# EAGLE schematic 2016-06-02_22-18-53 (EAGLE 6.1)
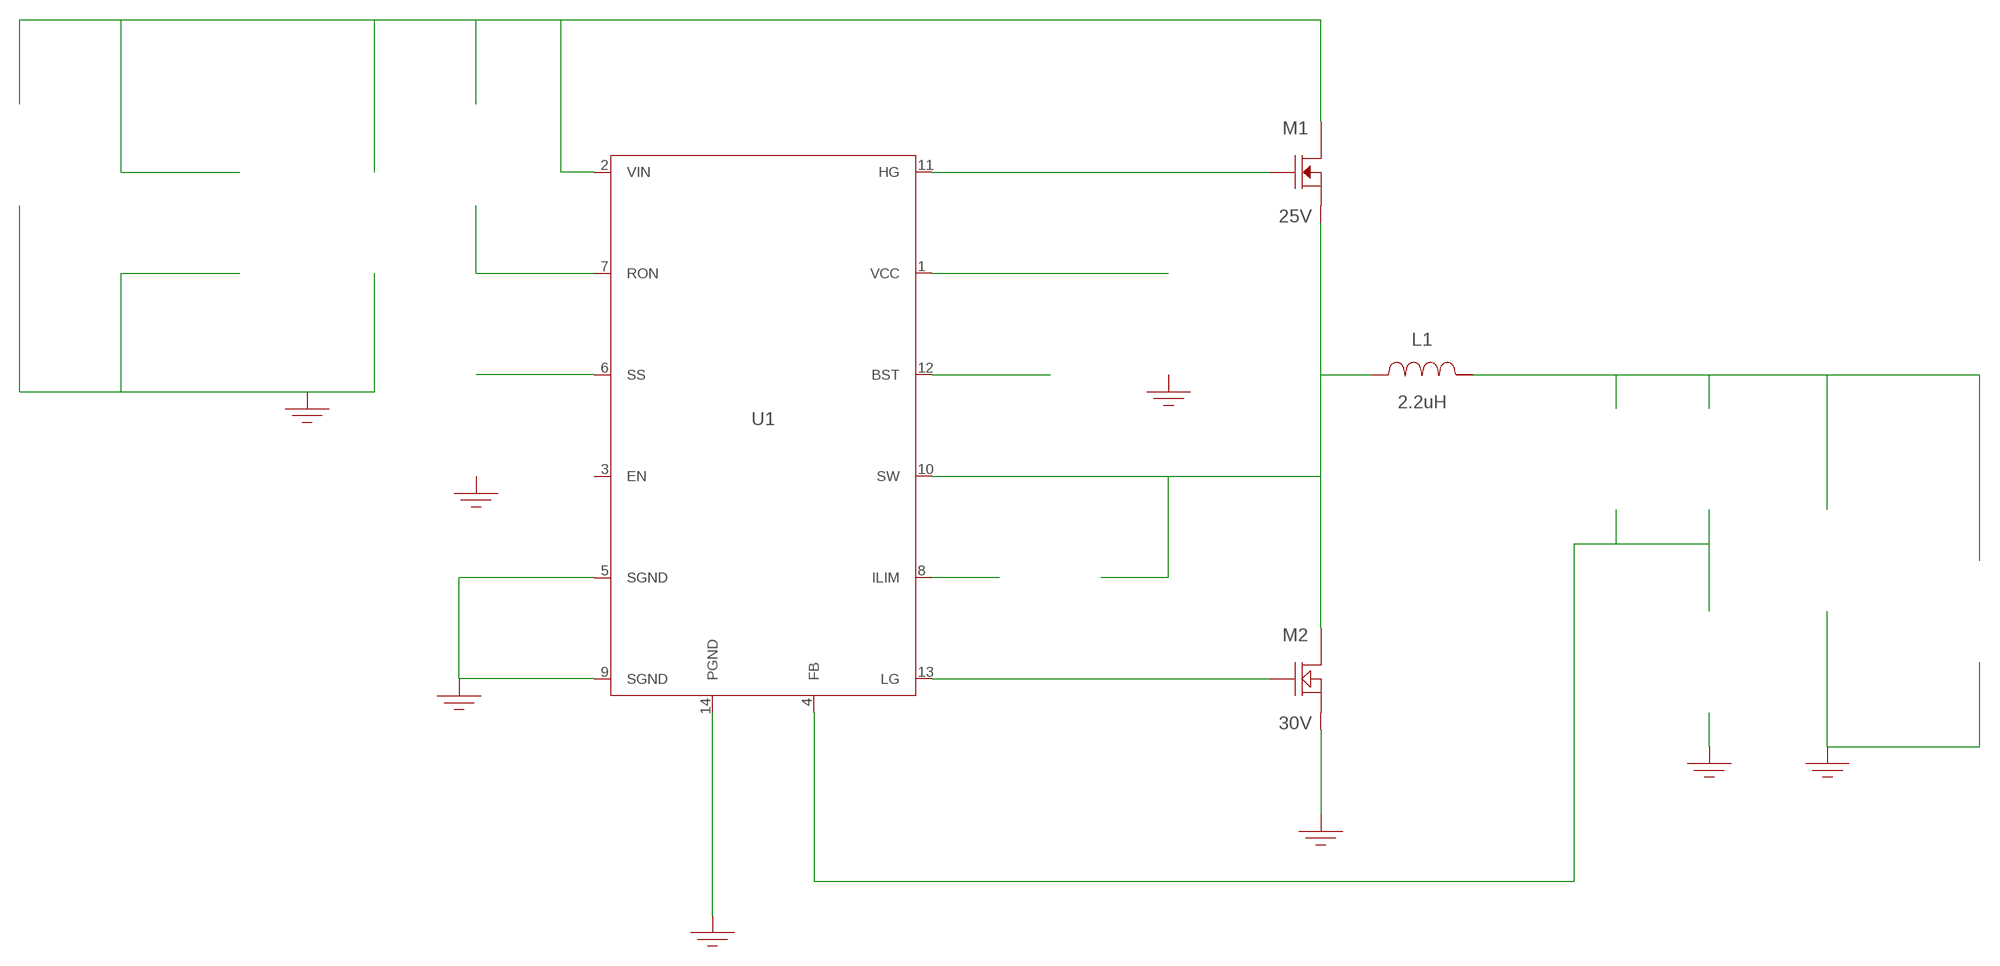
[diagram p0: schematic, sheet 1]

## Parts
CBST  470nF  EMK212B7474KD-TEMK212B7474KD-T  [0805]  (not placed on a sheet)
CBYP  100nF  08053C104KAT2A08053C104KAT2A  [0805]  (not placed on a sheet)
CFF  470pF  C0805C471K5RACTUC0805C471K5RACTU  [0805]  (not placed on a sheet)
CIN  22uF  GRM32ER61E226KE15LGRM32ER61E226KE15L  [1210]  (not placed on a sheet)
CIN_2  22uF  GRM32ER61E226KE15LGRM32ER61E226KE15L  [1210]  (not placed on a sheet)
COUT  220uF  6SVPE220MW6SVPE220MW  [CAPSMT_62_E61]  (not placed on a sheet)
CSS  15nF  CC0805KRX7R9BB153CC0805KRX7R9BB153  [0805]  (not placed on a sheet)
CVCC  1uF  EMK212B7105KG-TEMK212B7105KG-T  [0805]  (not placed on a sheet)
GND1  WB_GND  WB_GNDWB_GND  [WB_GND]
GND2  WB_GND  WB_GNDWB_GND  [WB_GND]
GND3  WB_GND  WB_GNDWB_GND  [WB_GND]
GND4  WB_GND  WB_GNDWB_GND  [WB_GND]
GND5  WB_GND  WB_GNDWB_GND  [WB_GND]
GND6  WB_GND  WB_GNDWB_GND  [WB_GND]
GND7  WB_GND  WB_GNDWB_GND  [WB_GND]
GND8  WB_GND  WB_GNDWB_GND  [WB_GND]
IOUT  WB_CURRENT_LOAD  WB_CURRENT_LOADWB_CURRENT_LOAD  [WB_CURRENT_LOAD]  (not placed on a sheet)
L1  2.2uH  SRP1270-2R2MSRP1270-2R2M  [SRP1270]
M1  25V  CSD16342Q5ACSD16342Q5A  [TRANS_NexFET_Q5A]
M2  30V  CSD17577Q5ACSD17577Q5A  [TRANS_NexFET_Q5A]
RFB1  10k  ERJ-6ENF1002VERJ-6ENF1002V  [0805]  (not placed on a sheet)
RFB2  73.2k  ERJ-6ENF7322VERJ-6ENF7322V  [0805]  (not placed on a sheet)
RILIM  1.05k  ERJ-6ENF1051VERJ-6ENF1051V  [0805]  (not placed on a sheet)
RON  100k  ERJ-6ENF1003VERJ-6ENF1003V  [0805]  (not placed on a sheet)
U1  LM3150MH/NOPB  LM3150MH/NOPBLM3150MH/NOPB  [MXA14A]
VIN  WB_BATTERY  WB_BATTERYWB_BATTERY  [WB_BATTERY]  (not placed on a sheet)

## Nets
0: Cbyp.2@2 Cin.2@2 Cin_2.2@2 Cout.-@2 Css.2@2 Cvcc.2@2 GND1.1 GND2.1 GND3.1 GND4.1 GND5.1 GND6.1 GND7.1 GND8.1 Iout.-@2 M2.1(Source) M2.2(Source) M2.3(Source) Rfb1.2@2 U1.5(SGND) U1.9(SGND) U1.14(PGND) U1.15(DAP) Vin.-@2
1: Css.1@1 U1.6(SS)
2: Cbyp.1@1 Cin.1@1 Cin_2.1@1 M1.5(Drain) M1.6(Drain) M1.7(Drain) M1.8(Drain) M1.9(Drain) Ron.1@1 U1.2(VIN) Vin.+@1
3: Ron.2@2 U1.7(RON)
4: Cff.1@1 Cout.+@1 Iout.+@1 L1.2 Rfb2.1@1
5: Cff.2@2 Rfb1.1@1 Rfb2.2@2 U1.4(FB)
6: Cbst.2@2 L1.1 M1.1(Source) M1.2(Source) M1.3(Source) M2.5(Drain) M2.6(Drain) M2.7(Drain) M2.8(Drain) M2.9(Drain) Rilim.1@1 U1.10(SW)
7: M2.4(Gate) U1.13(LG)
8: M1.4(Gate) U1.11(HG)
9: Cbst.1@1 U1.12(BST)
10: Cvcc.1@1 U1.1(VCC)
11: Rilim.2@2 U1.8(ILIM)
Unconnected: CBST.1 CBST.2 CBYP.1 CBYP.2 CFF.1 CFF.2 CIN.1 CIN.2 CIN_2.1 CIN_2.2 COUT.1(+) COUT.2(-) CSS.1 CSS.2 CVCC.1 CVCC.2 IOUT.1(+) IOUT.2(-) RFB1.1 RFB1.2 RFB2.1 RFB2.2 RILIM.1 RILIM.2 RON.1 RON.2 U1.3(EN) VIN.1(+) VIN.2(-)

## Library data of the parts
CBST = AcceleratedDesigns_Lib:EMK212B7474KD-T; Cap: 4.7E-7; ESR: 0.0; IRMS: 0.0; Manufacturer_Name: Taiyo Yuden; Manufacturer_Part_Number: EMK212B7474KD-T; VDC: 16.0; Vendor: Taiyo Yuden
CBYP = AcceleratedDesigns_Lib:08053C104KAT2A; Cap: 1.0E-7; ESR: 0.28; IRMS: 0.0; Manufacturer_Name: AVX; Manufacturer_Part_Number: 08053C104KAT2A; VDC: 25.0; Vendor: AVX
CFF = AcceleratedDesigns_Lib:C0805C471K5RACTU; Cap: 4.7E-10; ESR: 0.688; IRMS: 0.213; Manufacturer_Name: Kemet; Manufacturer_Part_Number: C0805C471K5RACTU; VDC: 50.0; Vendor: Kemet
CIN CIN_2 = AcceleratedDesigns_Lib:GRM32ER61E226KE15L; Cap: 2.2E-5; ESR: 0.0020; IRMS: 0.0; Manufacturer_Name: MuRata; Manufacturer_Part_Number: GRM32ER61E226KE15L; VDC: 25.0; Vendor: MuRata
COUT = AcceleratedDesigns_Lib:6SVPE220MW; Cap: 2.2E-4; Datasheet_URL: http://industrial.panasonic.com/www%2Ddata/pdf/AAB8000/AAB8000CE2.pdf; ESR: 0.015; IRMS: 3.15; Manufacturer_Name: Panasonic; Manufacturer_Part_Number: 6SVPE220MW; VDC: 6.3; Vendor: Panasonic
CSS = AcceleratedDesigns_Lib:CC0805KRX7R9BB153; Cap: 1.5E-8; ESR: 0.0; IRMS: 0.0; Manufacturer_Name: Yageo America; Manufacturer_Part_Number: CC0805KRX7R9BB153; VDC: 50.0; Vendor: Yageo America
CVCC = AcceleratedDesigns_Lib:EMK212B7105KG-T; Cap: 1.0E-6; ESR: 0.0; IRMS: 0.0; Manufacturer_Name: Taiyo Yuden; Manufacturer_Part_Number: EMK212B7105KG-T; VDC: 16.0; Vendor: Taiyo Yuden
GND1-GND8 = AcceleratedDesigns_Lib:WB_GND; Manufacturer_Name: WB_GND; Manufacturer_Part_Number: WB_GND; PowerPortType: POWER_GROUND; Value: Value
IOUT = AcceleratedDesigns_Lib:WB_CURRENT_LOAD; Manufacturer_Name: WB_CURRENT_LOAD; Manufacturer_Part_Number: WB_CURRENT_LOAD; PowerPortType: POWER_GROUND; Value: Value
L1 = AcceleratedDesigns_Lib:SRP1270-2R2M; DCR: 0.0042; IDC: 22.0; L: 2.2E-6; Manufacturer_Name: Bourns; Manufacturer_Part_Number: SRP1270-2R2M; Vendor: Bourns
M1 = AcceleratedDesigns_Lib:CSD16342Q5A; Datasheet_URL: http://www.ti.com/lit/ds/symlink/csd16342q5a.pdf; IdsMax: 100.0; Manufacturer_Name: Texas Instruments; Manufacturer_Part_Number: CSD16342Q5A; QgTyp: 6.8; Quantity: 1; Rdson45: 0.0043; VdsMax: 25.0; Vendor: Texas Instruments
M2 = AcceleratedDesigns_Lib:CSD17577Q5A; Datasheet_URL: http://www.ti.com/lit/ds/symlink/CSD17577Q5A.pdf; IdsMax: 22.0A; Manufacturer_Name: Texas Instruments; Manufacturer_Part_Number: CSD17577Q5A; QgTyp: 13.0nC; Quantity: 1; Rdsonat10V: 0.0035Ohm; VdsMax: 30.0V; Vendor: Texas Instruments
RFB1 = AcceleratedDesigns_Lib:ERJ-6ENF1002V; Manufacturer_Name: Panasonic; Manufacturer_Part_Number: ERJ-6ENF1002V; Power: 0.125; Resistance: 10000.0; Tolerance: 1.0; Vendor: Panasonic
RFB2 = AcceleratedDesigns_Lib:ERJ-6ENF7322V; Manufacturer_Name: Panasonic; Manufacturer_Part_Number: ERJ-6ENF7322V; Power: 0.125; Resistance: 73200.0; Tolerance: 1.0; Vendor: Panasonic
RILIM = AcceleratedDesigns_Lib:ERJ-6ENF1051V; Manufacturer_Name: Panasonic; Manufacturer_Part_Number: ERJ-6ENF1051V; Power: 0.125; Resistance: 1050.0; Tolerance: 1.0; Vendor: Panasonic
RON = AcceleratedDesigns_Lib:ERJ-6ENF1003V; Manufacturer_Name: Panasonic; Manufacturer_Part_Number: ERJ-6ENF1003V; Power: 0.125; Resistance: 100000.0; Tolerance: 1.0; Vendor: Panasonic
U1 = AcceleratedDesigns_Lib:LM3150MH/NOPB; Datasheet_URL: http://www.ti.com/product/lm3150; Frequency: 1000000.0; Imax: 12.0; Manufacturer_Name: Texas Instruments; Manufacturer_Part_Number: LM3150MH/NOPB; Mktg_Package: NA; NSID: LM3150MH/NOPB; Package: NA; Vendor: Texas Instruments
VIN = AcceleratedDesigns_Lib:WB_BATTERY; Manufacturer_Name: WB_BATTERY; Manufacturer_Part_Number: WB_BATTERY; PowerPortType: POWER_GROUND; Value: Value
